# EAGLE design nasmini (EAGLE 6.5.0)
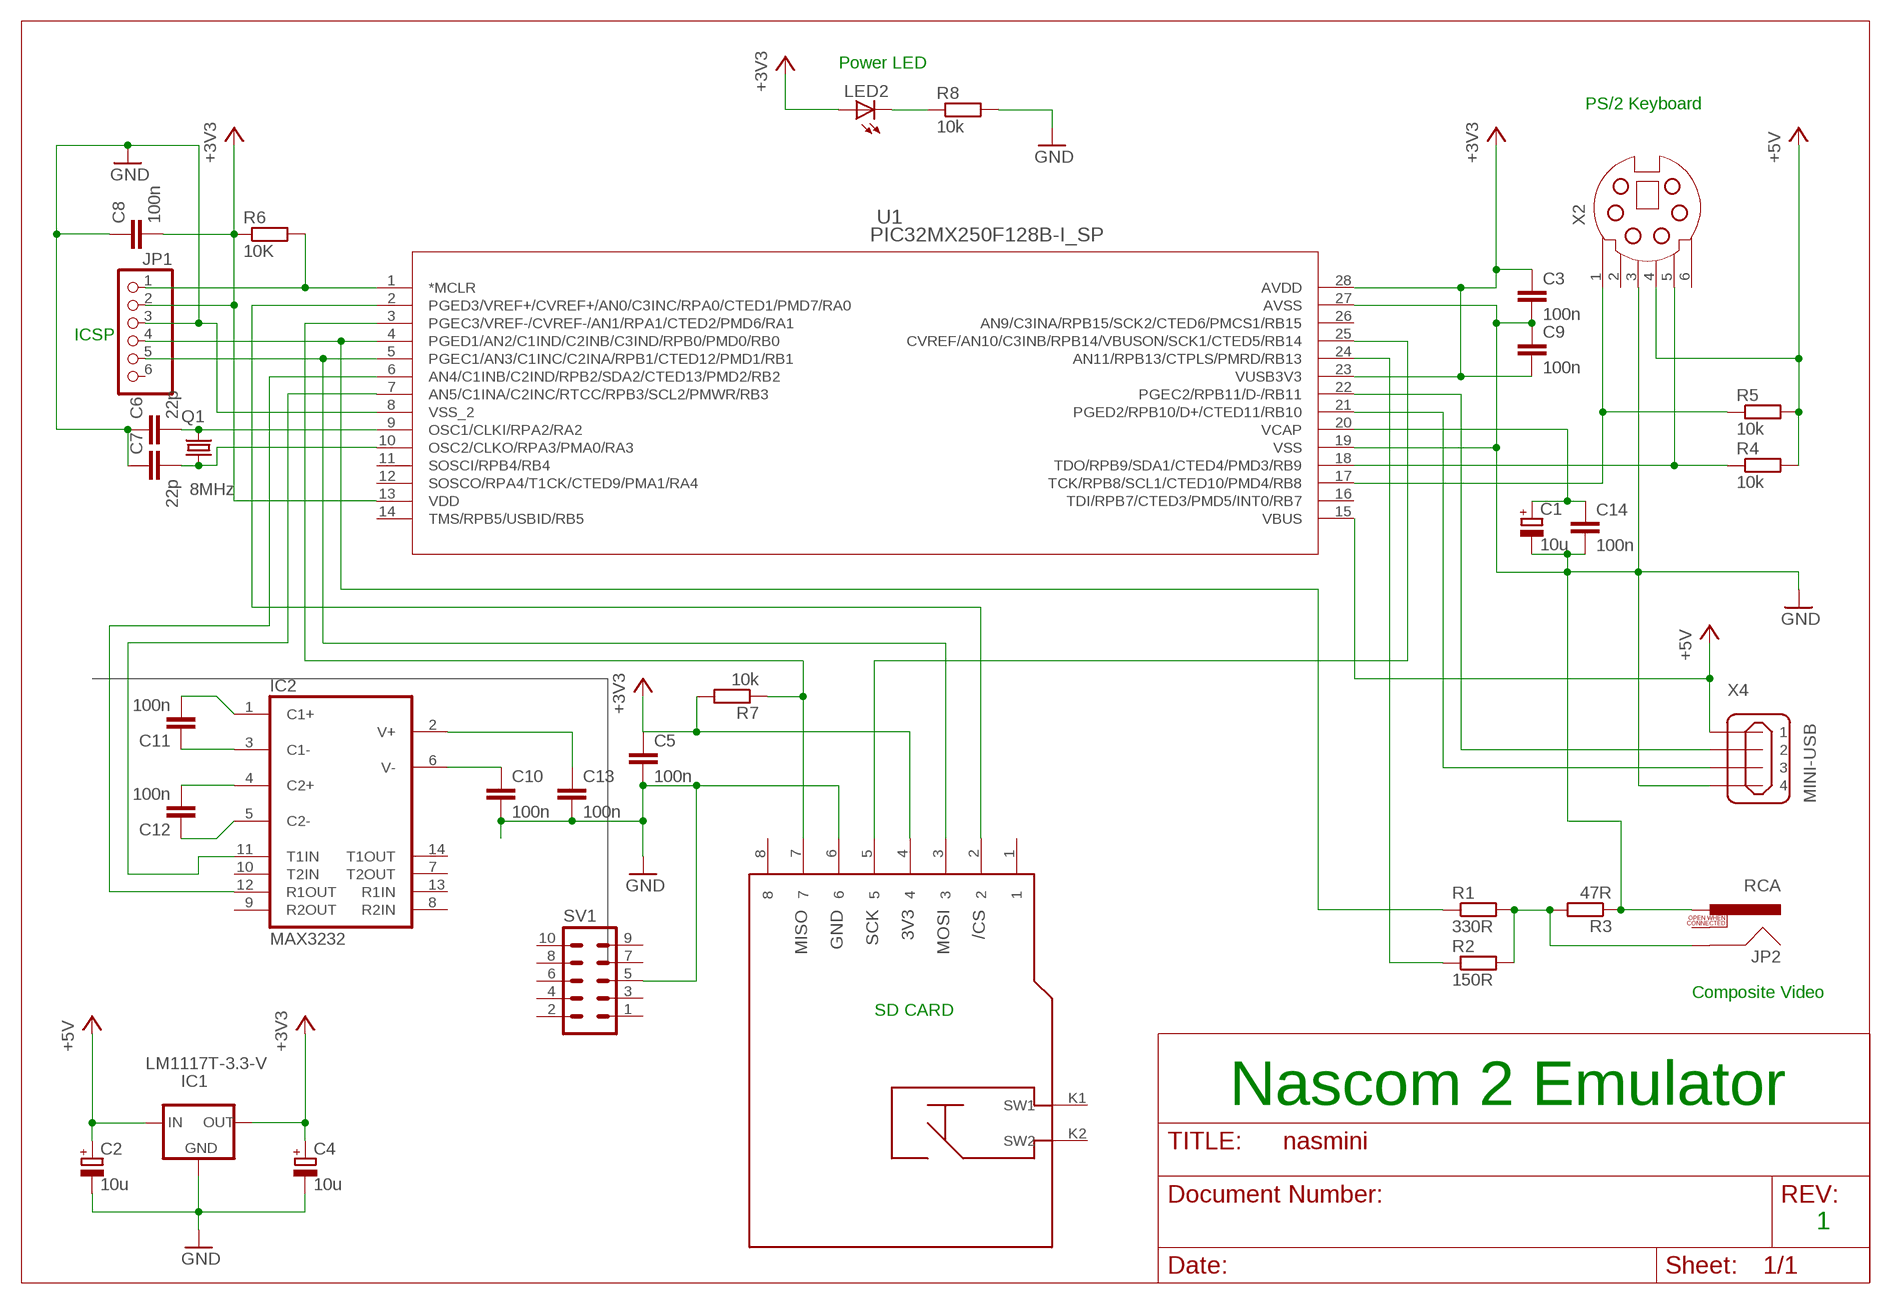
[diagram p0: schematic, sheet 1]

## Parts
C1  10u  CPOL-EUE2.5-5  [E2,5-5]
C2  10u  CPOL-EUE2.5-5  [E2,5-5]
C3  100n  C-EU025-025X050  [C025-025X050]
C4  10u  CPOL-EUE2.5-5  [E2,5-5]
C5  100n  C-EU025-025X050  [C025-025X050]
C6  22p  C-EU025-025X050  [C025-025X050]
C7  22p  C-EU025-025X050  [C025-025X050]
C8  100n  C-EU025-025X050  [C025-025X050]
C9  100n  C-EU025-025X050  [C025-025X050]
C10  100n  C-EU025-025X050  [C025-025X050]
C11  100n  C-EU025-025X050  [C025-025X050]
C12  100n  C-EU025-025X050  [C025-025X050]
C13  100n  C-EU025-025X050  [C025-025X050]
C14  100n  C-EU025-025X050  [C025-025X050]
IC1  LM1117T-3.3-V  [TO220V]
IC2  MAX3232  MAX232  [DIL16]
JP1  PINHD-1X6  [1X06]
JP2  RCA  [RCA]
LED2  LED3MM  [LED3MM]
Q1  8MHz  CRYSTALHC49S  [HC49/S]
R1  330R  R-EU_0207/7  [0207/7]
R2  150R  R-EU_0207/7  [0207/7]
R3  47R  R-EU_0207/7  [0207/7]
R4  10k  R-EU_0207/7  [0207/7]
R5  10k  R-EU_0207/7  [0207/7]
R6  10K  R-EU_0207/7  [0207/7]
R7  10k  R-EU_0207/7  [0207/7]
R8  10k  R-EU_0207/7  [0207/7]
SV1  MA05-2  [MA05-2]
U1  PIC32MX250F128B-I_SP  [SPDIP28_300MC]
X2  MDSSV-F06  [SSV-BC06]
X4  MINI-USB  MINI-USB_SHIELD4P-85-32006-201-1  [85-32006-201-1]
X5  MICRO-SD  [MICRO-SD]

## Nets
+3V3: C3.1 C4.+ C8.2 C9.2 IC1.2(OUT) JP1.2 LED2.A R6.1 R7.2 U1.13(VDD) U1.23(VUSB3V3) U1.28(AVDD) X5.4
+5V: C2.+ IC1.3(IN) R4.2 R5.2 U1.15(VBUS) X2.4 X4.1
GND: C1.- C2.- C3.2 C4.- C5.2 C6.1 C7.1 C8.1 C9.1 C10.2 C13.2 C14.2 IC1.1(GND) JP1.3 JP2.PIN R3.1 R8.2 SV1.5 U1.8(VSS_2) U1.19(VSS) U1.27(AVSS) X2.3 X4.4 X5.6
N$1: R5.1 U1.17(TCK/RPB8/SCL1/CTED10/PMD4/RB8) X2.1
N$2: R4.1 U1.18(TDO/RPB9/SDA1/CTED4/PMD3/RB9) X2.5
N$3: R2.1 U1.24(AN11/RPB13/CTPLS/PMRD/RB13)
N$5: JP2.SHELL R1.2 R2.2 R3.2
N$6: JP1.1 R6.2 U1.1(*MCLR)
N$7: C1.+ C14.1 U1.20(VCAP)
N$8: JP1.4 R1.1 U1.4(PGED1/AN2/C1IND/C2INB/C3IND/RPB0/PMD0/RB0)
N$10: U1.25(CVREF/AN10/C3INB/RPB14/VBUSON/SCK1/CTED5/RB14) X5.5
N$11: U1.2(PGED3/VREF+/CVREF+/AN0/C3INC/RPA0/CTED1/PMD7/RA0) X5.2
N$12: R7.1 U1.3(PGEC3/VREF-/CVREF-/AN1/RPA1/CTED2/PMD6/RA1) X5.7
N$13: JP1.5 U1.5(PGEC1/AN3/C1INC/C2INA/RPB1/CTED12/PMD1/RB1) X5.3
N$14: U1.21(PGED2/RPB10/D+/CTED11/RB10) X4.3
N$15: C7.2 Q1.1 U1.10(OSC2/CLKO/RPA3/PMA0/RA3)
N$16: C6.2 Q1.2 U1.9(OSC1/CLKI/RPA2/RA2)
N$17: U1.22(PGEC2/RPB11/D-/RB11) X4.2
N$20: C13.1 IC2.2(V+)
N$21: C10.1 IC2.6(V-)
N$22: C12.1 IC2.5(C2-)
N$23: C12.2 IC2.4(C2+)
N$24: C11.1 IC2.3(C1-)
N$25: C11.2 IC2.1(C1+)
N$26: IC2.11(T1IN) U1.7(AN5/C1INA/C2INC/RTCC/RPB3/SCL2/PMWR/RB3)
N$27: IC2.12(R1OUT) U1.6(AN4/C1INB/C2IND/RPB2/SDA2/CTED13/PMD2/RB2)
N$28: LED2.K(C) R8.1
Unconnected: C5.1 IC2.7(T2OUT) IC2.8(R2IN) IC2.9(R2OUT) IC2.10(T2IN) IC2.13(R1IN) IC2.14(T1OUT) JP1.6 JP2.SWITCH SV1.1 SV1.2 SV1.3 SV1.4 SV1.6 SV1.7 SV1.8 SV1.9 SV1.10 U1.11(SOSCI/RPB4/RB4) U1.12(SOSCO/RPA4/T1CK/CTED9/PMA1/RA4) U1.14(TMS/RPB5/USBID/RB5) U1.16(TDI/RPB7/CTED3/PMD5/INT0/RB7) U1.26(AN9/C3INA/RPB15/SCK2/CTED6/PMCS1/RB15) X2.2 X2.6 X4.M1(S1) X4.M2(S2) X5.1 X5.8 X5.K1(SW1) X5.K2(SW2)

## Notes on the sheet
- Power LED
- PS/2 Keyboard
- ICSP
- Composite Video
- SD CARD
- Nascom 2 Emulator
- 1

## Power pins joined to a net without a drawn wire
GND: IC2.15(GND)
VCC: IC2.16(VCC)

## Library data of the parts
C1 C2 C4 = rcl:CPOL-EU: POLARIZED CAPACITOR, European symbol
C3 C5-C14 = rcl:C-EU: CAPACITOR, European symbol
IC1 = lm1117:LM1117T-*
IC2 = maxim:MAX232: RS232 TRANSEIVER; MF: MAXIM; MPN: MAX232ACPE+; OC_FARNELL: 9723773; OC_NEWARK: 68K4544
JP1 = pinhead:PINHD-1X6: PIN HEADER
JP2 = SparkFun-Connectors:RCA
LED2 = led:LED: LED
Q1 = crystal:CRYSTAL: CRYSTAL; OC_FARNELL: 1667008; OC_NEWARK: unknown
R1-R8 = rcl:R-EU_: RESISTOR, European symbol
SV1 = con-lstb:MA05-2: PIN HEADER; OC_FARNELL: unknown; OC_NEWARK: unknown
U1 = pic32mx12:PIC32MX250F128B-I_SP
X2 = con-yamaichi:MDSSV-F06: YAMAICHI CONNECTOR; OC_FARNELL: unknown; OC_NEWARK: unknown
X4 = con-cypressindustries:MINI-USB_SHIELD4P-: MINI USB 4 Pol. Source: www.cypressindustries.com; OC_FARNELL: unknown; OC_NEWARK: unknown
X5 = welectronic:MICRO-SD

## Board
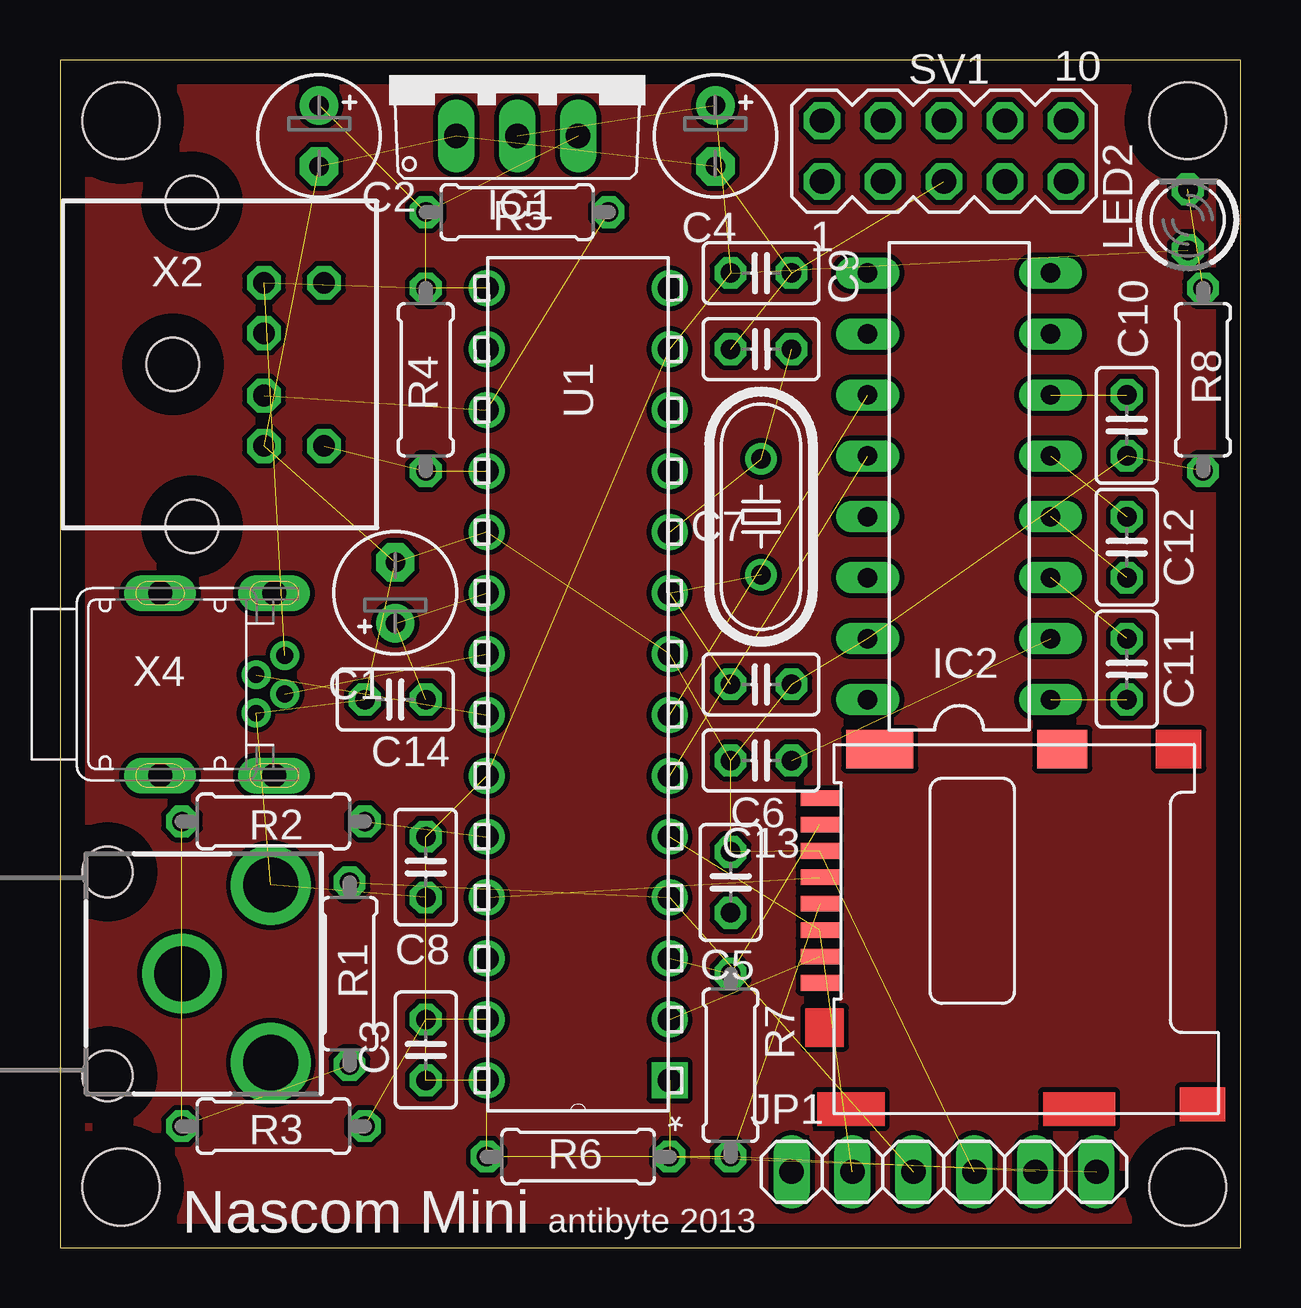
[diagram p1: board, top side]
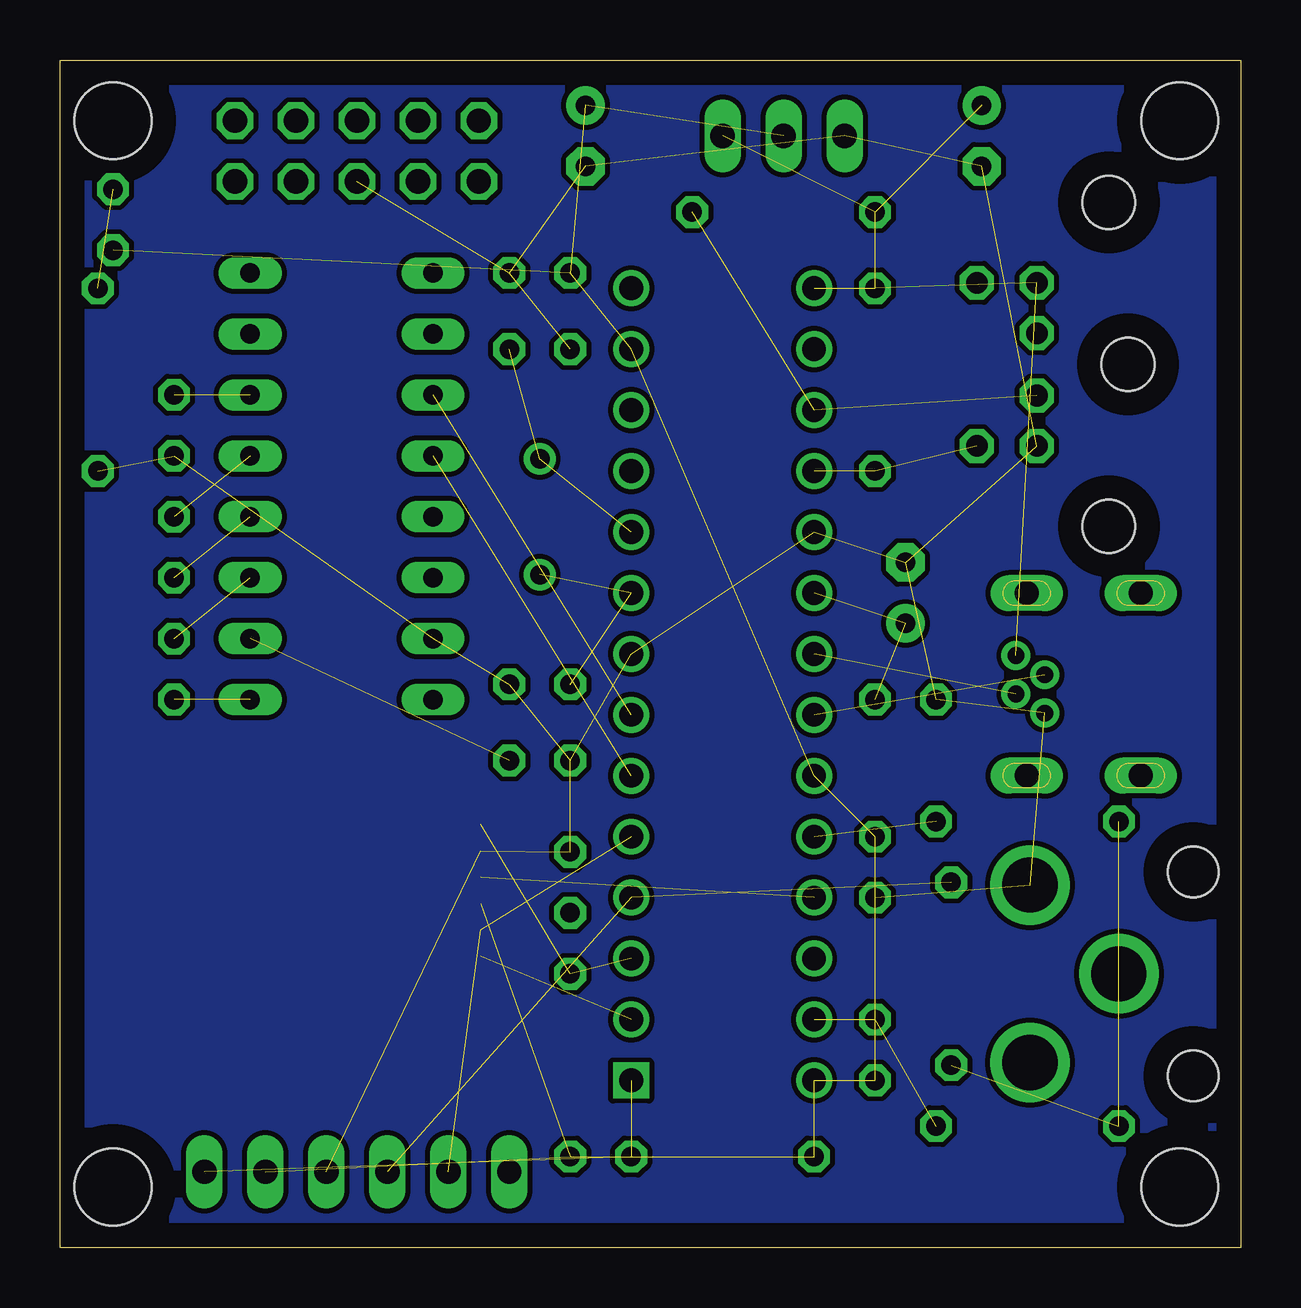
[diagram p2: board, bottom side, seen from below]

Size 49.2 x 49.52 mm. Coordinates in mm from the lower left corner, seen from the top.
Outline: 0,0 49.2,0 49.2,49.52 0,49.52 0,0
Copper layers (1*16): Top 0.035mm / dielectric 1.5mm / Bottom 0.035mm
Design rules "default *": minimum track width 8mil, minimum drill 24mil, track to track 8mil, track to pad 8mil, pad to pad 8mil, via to via 8mil, smd to smd 8mil, copper to edge 40mil, drill to drill 8mil, minimum pad ring 10mil, minimum via ring 8mil, stop-mask expansion 4mil, vias tented up to drill 0mil, thermal gap 10mil
Holes 3.2 mm at 2.54,2.54 2.54,46.99 46.99,2.54 46.99,46.99

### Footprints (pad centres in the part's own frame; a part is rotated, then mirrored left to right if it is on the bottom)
E2,5-5 = drill 0.813 pad 1.6: + -1.27,0 | drill 0.813 pad 1.6 octagon: - 1.27,0
C025-025X050 = drill 0.813 octagon: 1 -1.27,0; 2 1.27,0
TO220V = drill 1.016 long: 1 -2.54,-2.54; 2 0,-2.54; 3 2.54,-2.54
DIL16 = drill 0.813 long: 1 -8.89,-3.81; 2 -6.35,-3.81; 3 -3.81,-3.81; 4 -1.27,-3.81; 5 1.27,-3.81; 6 3.81,-3.81; 7 6.35,-3.81; 8 8.89,-3.81; 9 8.89,3.81; 10 6.35,3.81; 11 3.81,3.81; 12 1.27,3.81; 13 -1.27,3.81; 14 -3.81,3.81; 15 -6.35,3.81; 16 -8.89,3.81
1X06 = drill 1.016 long: 1 -6.35,0; 2 -3.81,0; 3 -1.27,0; 4 1.27,0; 5 3.81,0; 6 6.35,0
RCA = drill 2.3: PIN 3.7,3.7; SHELL 0,0; SWITCH 3.7,-3.7 | hole 2.1: -3.1,4.25; -3.1,-4.25
LED3MM = drill 0.813 octagon: A -1.27,0; K 1.27,0
HC49/S = drill 0.813: 1 -2.413,0; 2 2.413,0
0207/7 = drill 0.813 octagon: 1 -3.81,0; 2 3.81,0
MA05-2 = drill 1.016 octagon: 1 -5.08,-1.27; 2 -5.08,1.27; 3 -2.54,-1.27; 4 -2.54,1.27; 5 0,-1.27; 6 0,1.27; 7 2.54,-1.27; 8 2.54,1.27; 9 5.08,-1.27; 10 5.08,1.27
SPDIP28_300MC = drill 0.991 square: 1 -7.62,33.02 | drill 0.991: 2 -7.62,30.48; 3 -7.62,27.94; 4 -7.62,25.4; 5 -7.62,22.86; 6 -7.62,20.32; 7 -7.62,17.78; 8 -7.62,15.24; 9 -7.62,12.7; 10 -7.62,10.16; 11 -7.62,7.62; 12 -7.62,5.08; 13 -7.62,2.54; 14 -7.62,0; 15 0,0; 16 0,2.54; 17 0,5.08; 18 0,7.62; 19 0,10.16; 20 0,12.7; 21 0,15.24; 22 0,17.78; 23 0,20.32; 24 0,22.86; 25 0,25.4; 26 0,27.94; 27 0,30.48; 28 0,33.02
SSV-BC06 = drill 0.9 octagon: 1 1.3,8.5; 2 -1.3,8.5; 3 3.4,8.5; 4 -3.4,8.5; 5 3.4,11; 6 -3.4,11 | hole 2.2: -6.75,5.5; 0,4.7; 6.75,5.5
85-32006-201-1 = drill 0.7 pad 1.1: 1 -1.2,8.1; 2 -0.4,6.9; 3 0.4,8.1; 4 1.2,6.9 | drill 1 pad 1.4 long: M1 -3.8,2.9; M2 3.8,2.9; M3 -3.8,7.65; M4 3.8,7.65
MICRO-SD = smd 0.65 x 1.6: 1 -10.54,16.6; 2 -9.44,16.6; 3 -8.34,16.6; 4 -7.24,16.6; 5 -6.14,16.6; 6 -5.04,16.6; 7 -3.94,16.6; 8 -2.84,16.6 | smd 1.6 x 2.1: K1 -0.8,6.5 | smd 1.6 x 2.8: K2 -0.8,14.1

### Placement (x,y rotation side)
C1  13.97,27.3 90 top
C2  10.79,46.35 270 top
C3  15.24,8.26 90 top
C4  27.3,46.35 270 top
C5  27.94,15.24 90 top
C6  29.21,23.5 180 top
C7  29.21,37.47 0 top
C8  15.24,15.88 90 top
C9  29.21,40.64 180 top
C10  44.45,34.29 270 top
C11  44.45,24.13 270 top
C12  44.45,29.21 270 top
C13  29.21,20.32 180 top
C14  13.97,22.86 180 top
IC1  19.05,48.9 0 top
IC2  37.47,31.75 90 top
JP1  36.83,3.17 180 top
JP2  5.08,11.43 0 top
LED2  46.99,42.86 90 top
Q1  29.21,30.48 270 top
R1  12.06,11.43 270 top
R2  8.89,17.78 180 top
R3  8.89,5.08 180 top
R4  15.24,36.2 90 top
R5  19.05,43.18 180 top
R6  21.59,3.81 0 top
R7  27.94,7.62 270 top
R8  47.62,36.2 270 top
SV1  36.83,45.72 0 top
U1  17.78,40.01 180 top
X2  0,36.83 270 top
X4  1.27,23.5 270 top
X5  48.26,21.59 90 top

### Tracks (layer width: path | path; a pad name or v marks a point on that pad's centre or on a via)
+3V3  (12 unrouted)
+5V  (6 unrouted)
GND  (24 unrouted)
N$1  (2 unrouted)
N$2  (2 unrouted)
N$3  (1 unrouted)
N$5  (3 unrouted)
N$6  (2 unrouted)
N$7  (2 unrouted)
N$8  (2 unrouted)
N$10  (1 unrouted)
N$11  (1 unrouted)
N$12  (2 unrouted)
N$13  (2 unrouted)
N$14  (1 unrouted)
N$15  (2 unrouted)
N$16  (2 unrouted)
N$17  (1 unrouted)
N$18
  pour Top: 0,49.53 49.53,49.53 49.53,0 0,0
N$19
  pour Bottom: 0,49.53 49.53,49.53 49.53,0 0,0
N$20  (1 unrouted)
N$21  (1 unrouted)
N$22  (1 unrouted)
N$23  (1 unrouted)
N$24  (1 unrouted)
N$25  (1 unrouted)
N$26  (1 unrouted)
N$27  (1 unrouted)
N$28  (1 unrouted)

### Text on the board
tPlace: Nascom Mini | antibyte 2013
